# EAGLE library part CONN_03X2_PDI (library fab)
Multi connection point. Often used as Generic Header-pin footprint for 0.1 inch spaced/style header connections You can populate with any combo of single row headers, but if you'd like an exact match, check these: Header - 2x3 (Male, 0.1") (PRT-12807) Header - 2x3 (Female, 0.1") (PRT-13010) 2x3 Pin Shrouded Header (PRT-10877) On any of the 0.1 inch spaced packages, you can populate with these: Break Away Headers - Straight (PRT-00116) Break Away Male Headers - Right Angle (PRT-00553) Female Headers (PRT-00115) Break Away Headers - Machine Pin (PRT-00117) Break Away Female Headers - Swiss Machine Pin (PRT-00743) Special note: the shrouded connector mates well with our 3x2 ribbon cables: Ribbon Crimp Connector - 6-pin (2x3, Female) (PRT-10651) Ribbon Cable - 6 wire (15ft) (PRT-10646)
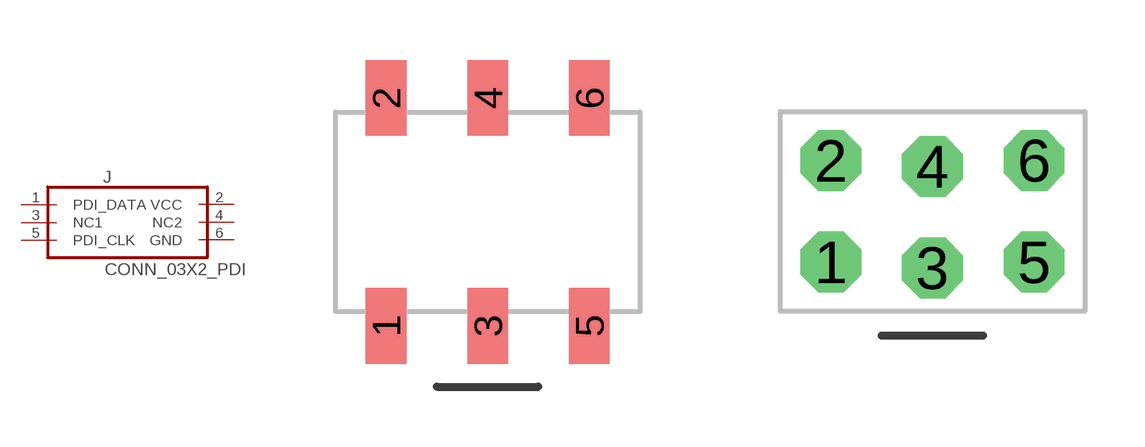
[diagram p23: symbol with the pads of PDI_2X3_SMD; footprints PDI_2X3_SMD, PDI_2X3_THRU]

Designator prefix J

## CONN_03X2_PDIFEMALE_SMD (PROD_ID: CONN-11290)  [PDI_2X3_SMD]
1  PDI_DATA
2  VCC
3  NC1
4  NC2
5  PDI_CLK
6  GND

## CONN_03X2_PDITHRU  [PDI_2X3_THRU]
Pads as for PDI_2X3_SMD

## Footprint PDI_2X3_SMD (pad centres in mm)
Surface Mount - 2x3 Specifications: Pin count:6 Pin pitch:2.54mm Example device(s): CONN_03x2
smd 1.02 x 1.9: 1 -2.54,-2.85; 2 -2.54,2.85; 3 0,-2.85; 4 0,2.85; 5 2.54,-2.85; 6 2.54,2.85

## Footprint PDI_2X3_THRU (pad centres in mm)
Surface Mount - 2x3 Specifications: Pin count:6 Pin pitch:2.54mm Example device(s): CONN_03x2
drill 1.016 octagon: 1 -2.54,-1.27; 2 -2.54,1.27; 3 0,-1.42; 4 0,1.12; 5 2.54,-1.27; 6 2.54,1.27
